| IBIS file was generated by Viper version: 2022.12.28
[IBIS Ver]   5.0
[Comment Char]   |_char
[File Name]   imxrt700_wlcsp256_v1_2.ibs
[File Rev]   1.2
[Date]   Sat Oct 12 16:54:56 2024
[Source]   NXP Viper 2022.12.28
[Notes]
[Disclaimer] IMPORTANT NOTICE
  This information is provided on an AS IS basis and without warranty.
  IN NO EVENT SHALL NXP BE LIABLE FOR INCIDENTAL OR CONSEQUENTIAL
  DAMAGES ARISING FROM USE OF THIS INFORMATION. THIS DISCLAIMER OF
  WARRANTY EXTENDS TO THE USER OF THE INFORMATION, AND TO THEIR CUSTOMERS
  OR USERS OF PRODUCTS  AND IS IN LIEU OF ALL WARRANTIES WHETHER EXPRESS,
  IMPLIED, OR STATUTORY, INCLUDING IMPLIED WARRANTIES OF MERCHANTABILITY
  OR FITNESS FOR PARTICULAR PURPOSE.
  NXP does not represent or warrant that the information furnished
  hereunder is free of infringement of any third party patents,
  copyrights, trade secrets, or other intellectual property rights.
  NXP does not represent or warrant that the information is free of
  defect, or that it meets any particular standard, requirements or need
  of the user of the infomation or their customers.
  NXP reserves the right to change the information in this file
  without notice.
   http://www.nxp.com
[Copyright]   (C) Copyright NXP 2004 - 2024, All Rights Reserved.
|   RT700_256WLCSP
[Component]   RT700_256WLCSP
[Manufacturer]   NXP
[Package]
| variable   typ   min   max
R_pkg   0.38753   0.03629   1.0051
L_pkg   6.781e-10   1.158e-10   1.519e-09
C_pkg   3.173e-13   1.393e-13   6.473e-13
[Pin] signal_name   model_name   R_pin   L_pin   C_pin
A1   VSS   GND   NA   NA   NA
A2   VSSA_0   GND   NA   NA   NA
A3   VDDA_1V8   POWER   NA   NA   NA
A4   PIO10_6   gpio   0.13675   2.891e-10 1.787e-13
A5   VDDIO_0_0   POWER   NA   NA   NA
A6   PIO8_0   gpio   0.10128   2.034e-10 1.632e-13
A7   VSS   GND   NA   NA   NA
A8   PIO8_17   gpio   0.077609  1.430e-10 1.682e-13
A9   VDD1   POWER   NA   NA   NA
A10   VSS_DCDC   GND   NA   NA   NA
A11   LX_DCDC   NC   0.072934  1.554e-10 4.207e-13
A12   VDD1V8_DCDC   POWER   NA   NA   NA
A13   VDD2_0   POWER   NA   NA   NA
A14   XTALOUT32KHZ   POWER   0.03629   1.158e-10 2.238e-13
A15   XTALIN32KHZ   POWER   0.040636  1.479e-10 1.539e-13
A16   VSS   GND   NA   NA   NA
B1   PIO10_1   gpio   0.11268   2.012e-10 1.856e-13
B2   PIO10_8   gpio   0.25366   4.256e-10 3.218e-13
B3   PIO10_9   gpio   0.27359   4.433e-10 2.674e-13
B4   PIO10_7   gpio   0.1909   3.677e-10 2.022e-13
B5   VDDIO_0_0   POWER   NA   NA   NA
B6   PIO8_1   gpio   0.24632   4.072e-10 2.348e-13
B7   PIO8_2   gpio   0.2466   4.307e-10 2.408e-13
B8   PIO8_3   gpio   0.26194   4.729e-10 2.265e-13
B9   VDD1   POWER   NA   NA   NA
B10   PMIC_I2C_SCL   gpio   0.1363   2.744e-10 2.610e-13
B11   PMIC_I2C_SDA   gpio   0.20546   3.788e-10 3.447e-13
B12   VDDN_0   POWER   NA   NA   NA
B13   VDD2_0   POWER   NA   NA   NA
B14   RESETN   reset   0.25137   4.556e-10 2.270e-13
B15   VSS   GND   NA   NA   NA
B16   VDD1V8_AO   POWER   NA   NA   NA
C1   PIO10_0   gpio   0.14455   3.381e-10 1.808e-13
C2   PIO10_2   gpio   0.31023   5.299e-10 2.460e-13
C3   VREF_LDO   POWER   0.19178   4.899e-10 3.872e-13
C4   PIO8_6   gpio   0.21434   3.975e-10 2.092e-13
C5   PIO8_4   gpio   0.26   4.578e-10 2.275e-13
C6   PIO8_5   gpio   0.31131   5.224e-10 2.495e-13
C7   PIO8_8   gpio   0.29036   5.135e-10 3.065e-13
C8   PIO8_14   gpio   0.30905   5.021e-10 2.593e-13
C9   PIO8_15   gpio   0.32803   5.435e-10 2.707e-13
C10   PIO8_16   gpio   0.31218   5.460e-10 3.216e-13
C11   VDD1V8   POWER   NA   NA   NA
C12   VDDIO_AO   POWER   NA   NA   NA
C13   PIO1_12   sd_mmc   0.41249   6.798e-10 2.980e-13
C14   PIO0_19   sd_mmc   0.36804   8.420e-10 2.904e-13
C15   PIO1_11   sd_mmc   0.29361   5.137e-10 2.434e-13
C16   PIO1_10   sd_mmc   0.19366   3.915e-10 2.045e-13
D1   VSS   GND   NA   NA   NA
D2   VSS   GND   NA   NA   NA
D3   PIO10_3   gpio   0.2779   4.801e-10 2.392e-13
D4   PIO10_4   gpio   0.37393   6.394e-10 3.540e-13
D5   PIO10_5   gpio   0.42222   7.120e-10 3.192e-13
D6   VSS   GND   NA   NA   NA
D7   PIO8_12   gpio   0.36657   6.101e-10 2.806e-13
D8   PIO8_19   gpio   0.37706   6.549e-10 2.737e-13
D9   PIO8_22   gpio   0.43698   6.959e-10 3.624e-13
D10   VSS   GND   NA   NA   NA
D11   PIO1_9   sd_mmc   0.56471   9.208e-10 3.737e-13
D12   VSS   GND   NA   NA   NA
D13   PIO0_22   sd_mmc   0.42184   8.887e-10 3.623e-13
D14   PIO1_7   sd_mmc   0.32252   5.518e-10 2.586e-13
D15   PIO1_14   sd_mmc   0.28704   5.084e-10 2.395e-13
D16   PIO1_13   sd_mmc   0.19496   4.560e-10 2.095e-13
E1   PIO8_31   gpio   0.099242  1.922e-10 1.767e-13
E2   PIO8_30   gpio   0.19738   3.274e-10 2.300e-13
E3   PIO8_23   gpio   0.3136   5.167e-10 2.581e-13
E4   VSS   GND   NA   NA   NA
E5   PIO10_12   gpio   0.75804   1.222e-09 5.015e-13
E6   PIO8_11   gpio   0.47056   7.592e-10 3.191e-13
E7   PIO8_13   gpio   0.48157   7.626e-10 3.248e-13
E8   PIO8_20   gpio   0.51434   8.462e-10 3.365e-13
E9   PIO8_21   gpio   0.51837   8.303e-10 4.456e-13
E10   VSS   GND   NA   NA   NA
E11   PIO1_17   sd_mmc   0.55531   9.071e-10 3.874e-13
E12   PIO1_18   sd_mmc   0.48338   7.978e-10 4.202e-13
E13   PIO0_21   sd_mmc   0.41051   7.837e-10 3.403e-13
E14   PIO1_8   sd_mmc   0.3817   6.499e-10 2.805e-13
E15   VDDIO_0_3   POWER   NA   NA   NA
E16   VDDIO_0_3   POWER   NA   NA   NA
F1   VDDIO_0_1   POWER   NA   NA   NA
F2   PIO7_20   sd_mmc   0.18104   3.085e-10 2.042e-13
F3   PIO7_18   sd_mmc   0.37712   6.858e-10 2.822e-13
F4   PIO8_7   gpio   0.42623   6.661e-10 3.029e-13
F5   PIO8_24   gpio   0.49513   7.774e-10 3.224e-13
F6   PIO8_10   gpio   0.61814   9.655e-10 3.879e-13
F7   PIO10_13   gpio   0.70021   1.138e-09 4.314e-13
F8   PIO8_18   gpio   0.56784   9.508e-10 4.232e-13
F9   PMIC_IRQN   gpio   0.83608   1.327e-09 5.498e-13
F10   PMIC_MODE0   reset   0.89726   1.411e-09 4.975e-13
F11   PMIC_MODE1   reset   0.80565   1.300e-09 5.347e-13
F12   PIO0_20   sd_mmc   0.57035   8.935e-10 3.634e-13
F13   VSS   GND   NA   NA   NA
F14   PIO0_10   sd_mmc   0.28933   6.076e-10 2.423e-13
F15   PIO0_11   sd_mmc   0.1742   3.289e-10 1.992e-13
F16   PIO0_13   sd_mmc   0.10129   2.336e-10 1.717e-13
G1   PIO7_17   sd_mmc   0.17417   3.209e-10 1.983e-13
G2   PIO7_19   sd_mmc   0.1371   2.597e-10 1.802e-13
G3   PIO7_22   sd_mmc   0.35574   6.151e-10 2.865e-13
G4   VSS   GND   NA   NA   NA
G5   VSS   GND   NA   NA   NA
G6   VSS   GND   NA   NA   NA
G7   PIO7_25   sd_mmc   0.66486   1.032e-09 4.557e-13
G8   PIO8_25   gpio   0.88469   1.286e-09 5.711e-13
G9   PIO8_26   gpio   1.0051   1.519e-09 6.473e-13
G10   PIO1_6   sd_mmc   0.75701   1.195e-09 4.596e-13
G11   PIO1_0   sd_mmc   0.68043   1.054e-09 4.124e-13
G12   PIO0_1   sd_mmc   0.70166   1.220e-09 4.435e-13
G13   PIO0_2   sd_mmc   0.53515   9.598e-10 4.137e-13
G14   PIO0_0   sd_mmc   0.44632   8.625e-10 3.698e-13
G15   PIO0_12   sd_mmc   0.17359   4.158e-10 2.157e-13
G16   PIO0_14   sd_mmc   0.15457   3.181e-10 1.859e-13
H1   VDD2_4   POWER   NA   NA   NA
H2   VDD2_4   POWER   NA   NA   NA
H3   PIO7_21   sd_mmc   0.34595   5.761e-10 2.655e-13
H4   PIO5_14   sd_mmc   0.49082   1.017e-09 3.304e-13
H5   PIO5_19   sd_mmc   0.53689   9.916e-10 3.569e-13
H6   PIO8_9   gpio   0.6146   1.058e-09 3.841e-13
H7   VSS   GND   NA   NA   NA
H8   VSS   GND   NA   NA   NA
H9   PIO1_16   sd_mmc   0.82672   1.355e-09 5.656e-13
H10   PIO1_15   sd_mmc   0.78323   1.218e-09 4.527e-13
H11   PIO0_31   sd_mmc   0.70274   1.065e-09 4.846e-13
H12   PIO2_5   gpiohv   0.60289   1.037e-09 4.548e-13
H13   PIO2_0   gpiohv   0.41333   7.895e-10 3.238e-13
H14   PIO0_3   sd_mmc   0.3059   5.393e-10 3.617e-13
H15   PIO0_4   sd_mmc   0.15334   3.228e-10 1.902e-13
H16   PIO0_5   sd_mmc   0.16717   3.221e-10 1.904e-13
J1   PIO5_7   sd_mmc   0.41555   1.091e-09 3.296e-13
J2   PIO5_8   sd_mmc   0.50551   1.143e-09 3.689e-13
J3   PIO5_13   sd_mmc   0.30602   6.296e-10 3.474e-13
J4   PIO5_12   sd_mmc   0.53561   1.017e-09 3.832e-13
J5   PIO5_17   sd_mmc   0.48571   8.234e-10 3.864e-13
J6   PIO5_16   sd_mmc   0.59762   1.018e-09 3.689e-13
J7   PIO7_13   sd_mmc   0.68627   1.092e-09 4.062e-13
J8   PIO7_14   sd_mmc   0.76954   1.236e-09 5.262e-13
J9   VSS   GND   NA   NA   NA
J10   VSS   GND   NA   NA   NA
J11   PIO2_7   gpiohv   0.6393   1.118e-09 4.567e-13
J12   PIO2_6   gpiohv   0.55407   1.014e-09 3.900e-13
J13   PIO2_1   gpiohv   0.36763   7.210e-10 2.830e-13
J14   PIO2_2   gpiohv   0.24667   5.044e-10 2.315e-13
J15   VDD2_1   POWER   NA   NA   NA
J16   VDD2_1   POWER   NA   NA   NA
K1   VSS   GND   NA   NA   NA
K2   PIO5_2   sd_mmc   0.4271   9.493e-10 3.314e-13
K3   PIO5_9   sd_mmc   0.50121   9.920e-10 3.429e-13
K4   PIO5_20   sd_mmc   0.30588   5.524e-10 2.512e-13
K5   PIO5_15   sd_mmc   0.48312   8.373e-10 3.210e-13
K6   PIO7_23   sd_mmc   0.69761   1.163e-09 4.944e-13
K7   PIO7_15   sd_mmc   0.69897   1.104e-09 4.883e-13
K8   PIO7_16   sd_mmc   0.76917   1.227e-09 5.301e-13
K9   PIO0_7   sd_mmc   0.72981   1.166e-09 5.163e-13
K10   PIO0_6   sd_mmc   0.65482   1.068e-09 3.942e-13
K11   VSS   GND   NA   NA   NA
K12   VSS   GND   NA   NA   NA
K13   VSS   GND   NA   NA   NA
K14   PIO2_3   gpiohv   0.31306   5.722e-10 2.504e-13
K15   PIO2_9   gpiohv   0.16009   3.292e-10 1.912e-13
K16   PIO2_4   gpiohv   0.09074   2.156e-10 1.719e-13
L1   PIO5_11   sd_mmc   0.12094   2.518e-10 1.686e-13
L2   PIO5_10   sd_mmc   0.17688   3.139e-10 1.959e-13
L3   PIO5_1   sd_mmc   0.45183   8.973e-10 3.200e-13
L4   VSS   GND   NA   NA   NA
L5   PIO5_18   sd_mmc   0.62213   1.097e-09 4.511e-13
L6   PIO4_16   sd_mmc   0.61165   9.961e-10 4.067e-13
L7   PIO4_20   sd_mmc   0.58001   9.394e-10 3.649e-13
L8   PIO4_15   sd_mmc   0.45771   9.030e-10 3.260e-13
L9   PIO2_15   gpiohv   0.81936   1.247e-09 5.791e-13
L10   PIO7_3   sd_mmc   0.5196   9.578e-10 3.685e-13
L11   PIO2_8   gpiohv   0.5468   8.757e-10 3.819e-13
L12   PIO3_1   sd_mmc   0.50015   9.172e-10 3.926e-13
L13   PIO3_0   sd_mmc   0.40545   8.453e-10 3.768e-13
L14   PIO2_11   gpiohv   0.24945   4.482e-10 2.797e-13
L15   PIO2_10   gpiohv   0.2305   4.251e-10 2.387e-13
L16   VSS   GND   NA   NA   NA
M1   VDDIO_5   POWER   NA   NA   NA
M2   VDDIO_5   POWER   NA   NA   NA
M3   PIO5_5   sd_mmc   0.31344   6.144e-10 3.040e-13
M4   PIO5_0   sd_mmc   0.51633   9.380e-10 4.394e-13
M5   PIO4_14   sd_mmc   0.63313   1.030e-09 4.152e-13
M6   PIO4_12   sd_mmc   0.59774   9.396e-10 4.334e-13
M7   VSS   GND   NA   NA   NA
M8   PIO4_18   sd_mmc   0.43599   7.061e-10 3.109e-13
M9   PIO4_13   sd_mmc   0.61049   1.253e-09 4.187e-13
M10   PIO7_2   sd_mmc   0.40861   7.129e-10 3.955e-13
M11   PIO7_10   sd_mmc   0.45254   7.314e-10 3.414e-13
M12   PIO7_11   sd_mmc   0.51297   8.439e-10 3.339e-13
M13   VSS   GND   NA   NA   NA
M14   PIO2_14   gpiohv   0.24447   4.100e-10 2.303e-13
M15   PIO2_12   gpiohv   0.1657   2.961e-10 1.950e-13
M16   PIO2_13   gpiohv   0.04096   1.219e-10 1.393e-13
N1   VDDN_1   POWER   NA   NA   NA
N2   PIO5_4   sd_mmc   0.20411   3.552e-10 2.054e-13
N3   PIO5_3   sd_mmc   0.32382   5.474e-10 3.178e-13
N4   PIO4_19   sd_mmc   0.9603   1.503e-09 5.281e-13
N5   VDDN_1   POWER   NA   NA   NA
N6   PIO4_17   sd_mmc   0.76943   1.188e-09 4.468e-13
N7   VSS   GND   NA   NA   NA
N8   PIO4_5   sd_mmc   0.49426   9.180e-10 4.061e-13
N9   PIO4_0   sd_mmc   0.40437   6.680e-10 2.906e-13
N10   PIO7_12   sd_mmc   0.32445   5.486e-10 3.015e-13
N11   VSS   GND   NA   NA   NA
N12   PIO7_4   sd_mmc   0.32249   5.018e-10 3.308e-13
N13   PIO7_5   sd_mmc   0.35599   5.987e-10 2.922e-13
N14   PIO3_2   sd_mmc   0.28346   4.998e-10 2.397e-13
N15   VDDIO_2   POWER   NA   NA   NA
N16   VDDIO_2   POWER   NA   NA   NA
P1   VDD3V3_USB   POWER   NA   NA   NA
P2   PIO5_6   sd_mmc   0.15909   2.857e-10 1.855e-13
P3   USB0_VBUS_DETECT   POWER   0.1483   3.668e-10 2.763e-13
P4   VSSA_1   GND   NA   NA   NA
P5   PIO4_7   sd_mmc   0.22615   4.118e-10 2.124e-13
P6   PIO4_9   sd_mmc   0.21753   3.937e-10 2.337e-13
P7   PIO4_1   sd_mmc   0.46201   9.070e-10 3.978e-13
P8   PIO4_3   sd_mmc   0.44768   9.337e-10 4.137e-13
P9   PIO4_4   sd_mmc   0.57763   1.189e-09 3.861e-13
P10   PIO7_1   sd_mmc   0.25603   4.403e-10 2.878e-13
P11   PIO7_9   sd_mmc   0.37344   5.754e-10 2.975e-13
P12   PIO7_8   sd_mmc   0.3285   5.441e-10 2.716e-13
P13   VDD1V1_MIPI_CAP   POWER   NA   NA   NA
P14   PIO3_3   sd_mmc   0.25231   4.761e-10 2.676e-13
P15   VDD1V8_MIPI   POWER   NA   NA   NA
P16   VDD2_2   POWER   NA   NA   NA
R1   USB0_DM   NC   0.16123   2.815e-10 2.266e-13
R2   VSS   GND   NA   NA   NA
R3   XTALINSYS   POWER   0.18893   3.113e-10 2.839e-13
R4   VDD1V8   POWER   NA   NA   NA
R5   PIO4_8   sd_mmc   0.33058   6.388e-10 2.600e-13
R6   PIO4_2   sd_mmc   0.13897   3.566e-10 1.855e-13
R7   PIO4_10   sd_mmc   0.24435   4.264e-10 2.118e-13
R8   VDDIO_4   POWER   NA   NA   NA
R9   PIO4_6   sd_mmc   0.39784   9.115e-10 3.063e-13
R10   PIO7_7   sd_mmc   0.16865   3.304e-10 2.059e-13
R11   PIO7_6   sd_mmc   0.21432   3.928e-10 2.092e-13
R12   VDDIO_0_2   POWER   NA   NA   NA
R13   MIPI_DSI_D0N   mipi   0.19251   3.136e-10 2.240e-13
R14   MIPI_DSI_CLKP   mipi   0.18085   2.881e-10 3.025e-13
R15   MIPI_DSI_CLKN   mipi   0.17021   2.839e-10 2.874e-13
R16   MIPI_DSI_D1N   mipi   0.19361   3.195e-10 2.671e-13
T1   VSS   GND   NA   NA   NA
T2   USB0_DP   NC   0.17527   2.824e-10 2.680e-13
T3   XTALOUTSYS   POWER   0.15146   2.707e-10 2.457e-13
T4   VDD1V8   POWER   NA   NA   NA
T5   VDDIO_4   POWER   NA   NA   NA
T6   PIO4_11   sd_mmc   0.25594   4.849e-10 2.402e-13
T7   VSS   GND   NA   NA   NA
T8   VDDIO_4   POWER   NA   NA   NA
T9   VSS   GND   NA   NA   NA
T10   VDD2_3   POWER   NA   NA   NA
T11   PIO7_0   sd_mmc   0.10901   2.453e-10 1.663e-13
T12   VDDIO_0_2   POWER   NA   NA   NA
T13   MIPI_DSI_D0P   mipi   0.16715   2.795e-10 2.114e-13
T14   VSS   GND   NA   NA   NA
T15   MIPI_DSI_D1P   mipi   0.1768   3.321e-10 2.478e-13
T16   VSS   GND   NA   NA   NA
[Pin Mapping]   pulldown_ref   pullup_ref
A1   VSS   NC
A2   VSSA_0   NC
A3   NC   VDDA_1V8
A4   VSS   NC
A5   NC   VDDIO_0_0
A6   VSS   NC
A7   VSS   NC
A8   VSS   NC
A9   NC   VDD1
A10   VSS_DCDC   NC
A11   NC   NC
A12   NC   VDD1V8_DCDC
A13   NC   VDD2_0
A14   NC   VDDIO_AO
A15   NC   VDDIO_AO
A16   VSS   NC
B1   VSS   NC
B2   VSS   NC
B3   VSS   NC
B4   VSS   NC
B5   NC   VDDIO_0_0
B6   VSS   NC
B7   VSS   NC
B8   VSS   NC
B9   NC   VDD1
B10   VSS   NC
B11   VSS   NC
B12   NC   VDDN_0
B13   NC   VDD2_0
B14   VSS   VDDIO_AO
B15   VSS   NC
B16   NC   VDD1V8_AO
C1   VSS   NC
C2   VSS   NC
C3   NC   VDDA_1V8
C4   VSS   NC
C5   VSS   NC
C6   VSS   NC
C7   VSS   NC
C8   VSS   NC
C9   VSS   NC
C10   VSS   NC
C11   NC   VDD1V8
C12   NC   VDDIO_AO
C13   VSS   NC
C14   VSS   NC
C15   VSS   NC
C16   VSS   NC
D1   VSS   NC
D2   VSS   NC
D3   VSS   NC
D4   VSS   NC
D5   VSS   NC
D6   VSS   NC
D7   VSS   NC
D8   VSS   NC
D9   VSS   NC
D10   VSS   NC
D11   VSS   NC
D12   VSS   NC
D13   VSS   NC
D14   VSS   NC
D15   VSS   NC
D16   VSS   NC
E1   VSS   NC
E2   VSS   NC
E3   VSS   NC
E4   VSS   NC
E5   VSS   NC
E6   VSS   NC
E7   VSS   NC
E8   VSS   NC
E9   VSS   NC
E10   VSS   NC
E11   VSS   NC
E12   VSS   NC
E13   VSS   NC
E14   VSS   NC
E15   NC   VDDIO_0_3
E16   NC   VDDIO_0_3
F1   NC   VDDIO_0_1
F2   VSS   NC
F3   VSS   NC
F4   VSS   NC
F5   VSS   NC
F6   VSS   NC
F7   VSS   NC
F8   VSS   NC
F9   VSS   VDDIO_AO
F10   VSS   VDDIO_AO
F11   VSS   VDDIO_AO
F12   VSS   NC
F13   VSS   NC
F14   VSS   NC
F15   VSS   NC
F16   VSS   NC
G1   VSS   NC
G2   VSS   NC
G3   VSS   NC
G4   VSS   NC
G5   VSS   NC
G6   VSS   NC
G7   VSS   NC
G8   VSS   NC
G9   VSS   NC
G10   VSS   NC
G11   VSS   NC
G12   VSS   NC
G13   VSS   NC
G14   VSS   NC
G15   VSS   NC
G16   VSS   NC
H1   NC   VDD2_4
H2   NC   VDD2_4
H3   VSS   NC
H4   VSS   VDDIO_5
H5   VSS   VDDIO_5
H6   VSS   NC
H7   VSS   NC
H8   VSS   NC
H9   VSS   NC
H10   VSS   NC
H11   VSS   NC
H12   VSS   VDDIO_2
H13   VSS   VDDIO_2
H14   VSS   NC
H15   VSS   NC
H16   VSS   NC
J1   VSS   VDDIO_5
J2   VSS   VDDIO_5
J3   VSS   VDDIO_5
J4   VSS   VDDIO_5
J5   VSS   VDDIO_5
J6   VSS   VDDIO_5
J7   VSS   NC
J8   VSS   NC
J9   VSS   NC
J10   VSS   NC
J11   VSS   VDDIO_2
J12   VSS   VDDIO_2
J13   VSS   VDDIO_2
J14   VSS   VDDIO_2
J15   NC   VDD2_1
J16   NC   VDD2_1
K1   VSS   NC
K2   VSS   VDDIO_5
K3   VSS   VDDIO_5
K4   VSS   VDDIO_5
K5   VSS   VDDIO_5
K6   VSS   NC
K7   VSS   NC
K8   VSS   NC
K9   VSS   NC
K10   VSS   NC
K11   VSS   NC
K12   VSS   NC
K13   VSS   NC
K14   VSS   VDDIO_2
K15   VSS   VDDIO_2
K16   VSS   VDDIO_2
L1   VSS   VDDIO_5
L2   VSS   VDDIO_5
L3   VSS   VDDIO_5
L4   VSS   NC
L5   VSS   VDDIO_5
L6   VSS   VDDIO_4
L7   VSS   VDDIO_4
L8   VSS   VDDIO_4
L9   VSS   VDDIO_2
L10   VSS   NC
L11   VSS   VDDIO_2
L12   VSS   NC
L13   VSS   NC
L14   VSS   VDDIO_2
L15   VSS   VDDIO_2
L16   VSS   NC
M1   NC   VDDIO_5
M2   NC   VDDIO_5
M3   VSS   VDDIO_5
M4   VSS   VDDIO_5
M5   VSS   VDDIO_4
M6   VSS   VDDIO_4
M7   VSS   NC
M8   VSS   VDDIO_4
M9   VSS   VDDIO_4
M10   VSS   NC
M11   VSS   NC
M12   VSS   NC
M13   VSS   NC
M14   VSS   VDDIO_2
M15   VSS   VDDIO_2
M16   VSS   VDDIO_2
N1   NC   VDDN_1
N2   VSS   VDDIO_5
N3   VSS   VDDIO_5
N4   VSS   VDDIO_4
N5   NC   VDDN_1
N6   VSS   VDDIO_4
N7   VSS   NC
N8   VSS   VDDIO_4
N9   VSS   VDDIO_4
N10   VSS   NC
N11   VSS   NC
N12   VSS   NC
N13   VSS   NC
N14   VSS   NC
N15   NC   VDDIO_2
N16   NC   VDDIO_2
P1   NC   VDD3V3_USB
P2   VSS   VDDIO_5
P3   NC   VDD3V3_USB
P4   VSSA_1   NC
P5   VSS   VDDIO_4
P6   VSS   VDDIO_4
P7   VSS   VDDIO_4
P8   VSS   VDDIO_4
P9   VSS   VDDIO_4
P10   VSS   NC
P11   VSS   NC
P12   VSS   NC
P13   NC   VDD1V1_MIPI_CAP
P14   VSS   NC
P15   NC   VDD1V8_MIPI
P16   NC   VDD2_2
R1   NC   NC
R2   VSS   NC
R3   NC   VDD1V8
R4   NC   VDD1V8
R5   VSS   VDDIO_4
R6   VSS   VDDIO_4
R7   VSS   VDDIO_4
R8   NC   VDDIO_4
R9   VSS   VDDIO_4
R10   VSS   NC
R11   VSS   NC
R12   NC   VDDIO_0_2
R13   VSS   VDD1V8_MIPI
R14   VSS   VDD1V8_MIPI
R15   VSS   VDD1V8_MIPI
R16   VSS   VDD1V8_MIPI
T1   VSS   NC
T2   NC   NC
T3   NC   VDD1V8
T4   NC   VDD1V8
T5   NC   VDDIO_4
T6   VSS   VDDIO_4
T7   VSS   NC
T8   NC   VDDIO_4
T9   VSS   NC
T10   NC   VDD2_3
T11   VSS   NC
T12   NC   VDDIO_0_2
T13   VSS   VDD1V8_MIPI
T14   VSS   NC
T15   VSS   VDD1V8_MIPI
T16   VSS   NC
[Diff Pin]  inv_pin  vdiff  tdelay_typ tdelay_min tdelay_max
R14   R15   NA   NA   NA   NA
T13   R13   NA   NA   NA   NA
T15   R16   NA   NA   NA   NA
|*   Model Selector   *
[Model Selector] gpio
io_crdrobe1dse0sre0   Derated range in cont mode, 5mA drive strength, without slew rate
io_crdrobe1dse0sre1   Derated range in cont mode, 5mA drive strength, with slew rate
io_crdrobe1dse1sre0   Derated range in cont mode, 10mA drive strength, without slew rate
io_crdrobe1dse1sre1   Derated range in cont mode, 10mA drive strength, with slew rate
io_crdr2obe1dse0sre0   Derated2 range in cont mode, 5mA drive strength, without slew rate
io_crdr2obe1dse0sre1   Derated2 range in cont mode, 5mA drive strength, with slew rate
io_crdr2obe1dse1sre0   Derated2 range in cont mode, 10mA drive strength, without slew rate
io_crdr2obe1dse1sre1   Derated2 range in cont mode, 10mA drive strength, with slew rate
io_lrobe1dse0sre0   low range mode, 5mA drive strength, without slew rate
io_lrobe1dse0sre1   low range mode, 5mA drive strength, with slew rate
io_lrobe1dse1sre0   low range mode, 10mA drive strength, without slew rate
io_lrobe1dse1sre1   low range mode, 10mA drive strength, with slew rate
[Model Selector] gpiohv
io_crnrobe1dse0sre0   Normal range in cont mode, 5mA drive strength, without slew rate
io_crnrobe1dse0sre1   Normal range in cont mode, 5mA drive strength, with slew rate
io_crnrobe1dse1sre0   Normal range in cont mode, 10mA drive strength, without slew rate
io_crnrobe1dse1sre1   Normal range in cont mode, 10mA drive strength, with slew rate
io_crdrobe1dse0sre0   Derated range in cont mode, 5mA drive strength, without slew rate
io_crdrobe1dse0sre1   Derated range in cont mode, 5mA drive strength, with slew rate
io_crdrobe1dse1sre0   Derated range in cont mode, 10mA drive strength, without slew rate
io_crdrobe1dse1sre1   Derated range in cont mode, 10mA drive strength, with slew rate
io_crdr2obe1dse0sre0   Derated2 range in cont mode, 5mA drive strength, without slew rate
io_crdr2obe1dse0sre1   Derated2 range in cont mode, 5mA drive strength, with slew rate
io_crdr2obe1dse1sre0   Derated2 range in cont mode, 10mA drive strength, without slew rate
io_crdr2obe1dse1sre1   Derated2 range in cont mode, 10mA drive strength, with slew rate
io_hrobe1dse0sre0   high range mode, 5mA drive strength, without slew rate
io_hrobe1dse0sre1   high range mode, 5mA drive strength, with slew rate
io_hrobe1dse1sre0   high range mode, 10mA drive strength, without slew rate
io_hrobe1dse1sre1   high range mode, 10mA drive strength, with slew rate
io_lrobe1dse0sre0   low range mode, 5mA drive strength, without slew rate
io_lrobe1dse0sre1   low range mode, 5mA drive strength, with slew rate
io_lrobe1dse1sre0   low range mode, 10mA drive strength, without slew rate
io_lrobe1dse1sre1   low range mode, 10mA drive strength, with slew rate
io_crnrobe1dse0sre0_5pct   Narrow range in cont mode, 5mA drive strength, without slew rate
io_crnrobe1dse0sre1_5pct   Narrow range in cont mode, 5mA drive strength, with slew rate
io_crnrobe1dse1sre0_5pct   Narrow range in cont mode, 10mA drive strength, without slew rate
io_crnrobe1dse1sre1_5pct   Narrow range in cont mode, 10mA drive strength, with slew rate
io_hrobe1dse0sre0_5pct   Narrow range in high range mode, 5mA drive strength, without slew rate
io_hrobe1dse0sre1_5pct   Narrow range in high range mode, 5mA drive strength, with slew rate
io_hrobe1dse1sre0_5pct   Narrow range in high range mode, 10mA drive strength, without slew rate
io_hrobe1dse1sre1_5pct   Narrow range in high range mode, 10mA drive strength, with slew rate
[Model Selector] mipi
MIPI_HS   MIPI DSI High Speed Mode
MIPI_LP   MIPI DSI Low Power Mode
[Model Selector] reset
io_rst_crdrobe1dse0sre0   Derated voltage range in cont mode, 5mA current drive strength, without slew rate
io_rst_crdrobe1dse0sre1   Derated voltage range in cont mode, 5mA current drive strength, with slew rate
io_rst_crdrobe1dse1sre0   Derated voltage range in cont mode, 10mA current drive strength, without slew rate
io_rst_crdrobe1dse1sre1   Derated voltage range in cont mode, 10mA current drive strength, with slew rate
io_rst_crdr2obe1dse0sre0   Derated2 voltage range in cont mode, 5mA current drive strength, without slew rate
io_rst_crdr2obe1dse0sre1   Derated2 voltage range in cont mode, 5mA current drive strength, with slew rate
io_rst_crdr2obe1dse1sre0   Derated2 voltage range in cont mode, 10mA current drive strength, without slew rate
io_rst_crdr2obe1dse1sre1   Derated2 voltage range in cont mode, 10mA current drive strength, with slew rate
io_rst_lrobe1dse0sre0   low range mode, 5mA current drive strength, without slew rate
io_rst_lrobe1dse0sre1   low range mode, 5mA current drive strength, with slew rate
io_rst_lrobe1dse1sre0   low range mode, 10mA current drive strength, without slew rate
io_rst_lrobe1dse1sre1   low range mode, 10mA current drive strength, with slew rate
[Model Selector] sd_mmc
io_nvldro0drz0   Normal voltage level DRIVE1=0 DRIVE0=0 1.8v voltage domain function mode with 100ohm transmitter drive
io_nvldro0drz1   Normal voltage level DRIVE1=0 DRIVE0=1 1.8v voltage domain function mode with 66ohm transmitter drive
io_nvldro1drz0   Normal voltage level DRIVE1=1 DRIVE0=0 1.8v voltage domain function mode with 50ohm transmitter drive
io_nvldro1drz1   Normal voltage level DRIVE1=1 DRIVE0=1 1.8v voltage domain function mode with 33ohm transmitter drive
io_lvldro0drz0   low voltage level DRIVE1=0 DRIVE0=0 1.2v voltage domain function mode with 100ohm transmitter drive
io_lvldro0drz1   low voltage level DRIVE1=0 DRIVE0=1 1.2v voltage domain function mode with 66ohm transmitter drive
io_lvldro1drz0   low voltage level DRIVE1=1 DRIVE0=0 1.2v voltage domain function mode with 50ohm transmitter drive
io_lvldro1drz1   low voltage level DRIVE1=1 DRIVE0=1 1.2v voltage domain function mode with 33ohm transmitter drive
| End [Component] RT700_256WLCSP
| Models and submodels in the file (50): MIPI_HS (Output), MIPI_LP (I/O), io_crdr2obe1dse0sre0 (I/O), io_crdr2obe1dse0sre1 (I/O), io_crdr2obe1dse1sre0 (I/O), io_crdr2obe1dse1sre1 (I/O), io_crdrobe1dse0sre0 (I/O), io_crdrobe1dse0sre1 (I/O), io_crdrobe1dse1sre0 (I/O), io_crdrobe1dse1sre1 (I/O), io_crnrobe1dse0sre0 (I/O), io_crnrobe1dse0sre0_5pct (I/O), io_crnrobe1dse0sre1 (I/O), io_crnrobe1dse0sre1_5pct (I/O), io_crnrobe1dse1sre0 (I/O), io_crnrobe1dse1sre0_5pct (I/O), io_crnrobe1dse1sre1 (I/O), io_crnrobe1dse1sre1_5pct (I/O), io_hrobe1dse0sre0 (I/O), io_hrobe1dse0sre0_5pct (I/O), io_hrobe1dse0sre1 (I/O), io_hrobe1dse0sre1_5pct (I/O), io_hrobe1dse1sre0 (I/O), io_hrobe1dse1sre0_5pct (I/O), io_hrobe1dse1sre1 (I/O), io_hrobe1dse1sre1_5pct (I/O), io_lrobe1dse0sre0 (I/O), io_lrobe1dse0sre1 (I/O), io_lrobe1dse1sre0 (I/O), io_lrobe1dse1sre1 (I/O), io_lvldro0drz0 (I/O), io_lvldro0drz1 (I/O), io_lvldro1drz0 (I/O), io_lvldro1drz1 (I/O), io_nvldro0drz0 (I/O), io_nvldro0drz1 (I/O), io_nvldro1drz0 (I/O), io_nvldro1drz1 (I/O), io_rst_crdr2obe1dse0sre0 (I/O), io_rst_crdr2obe1dse0sre1 (I/O), io_rst_crdr2obe1dse1sre0 (I/O), io_rst_crdr2obe1dse1sre1 (I/O), io_rst_crdrobe1dse0sre0 (I/O), io_rst_crdrobe1dse0sre1 (I/O), io_rst_crdrobe1dse1sre0 (I/O), io_rst_crdrobe1dse1sre1 (I/O), io_rst_lrobe1dse0sre0 (I/O), io_rst_lrobe1dse0sre1 (I/O), io_rst_lrobe1dse1sre0 (I/O), io_rst_lrobe1dse1sre1 (I/O)
